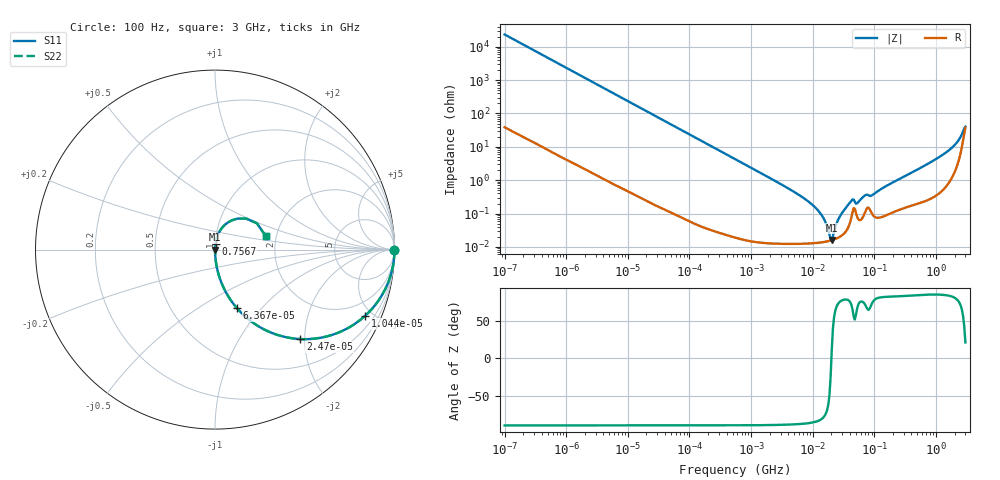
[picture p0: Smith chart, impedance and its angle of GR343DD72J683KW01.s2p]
!Murata Part Number: GR343DD72J683KW01
!These Parameters are Measured in Series Mode Connection
!Data Generated on Jan 08, 2026
!  o--ll--o
!Port1  Port2
!  o------o
!Operation Temp=25[degC], DC Bias Voltage=0[V]
!Freq. Start=100[Hz] Stop=3[GHz] 401[Steps]
# Hz S RI R 50
!Freq.(Hz) S11(Real) S11(Imag) S21(Real) S21(Imag) S12(Real) S12(Imag) S22(Real) S22(Imag)
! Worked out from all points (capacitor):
!   401 points, 100 Hz to 3 GHz, reference 50 ohm
!   read as one part in series: C = 68 nF near 109 Hz
!   lowest |Z| = 16.2 mohm at 20.36 MHz (marker M1)
!   series resonance near 20.1 MHz, so ESL is about 920 pH
!   S11 on the Smith chart (normalised r, x): 100 Hz: open; 10.44 kHz: 1.01, -4.51; 24.7 kHz: 1.00, -1.91; 63.67 kHz: 1.00, -0.74; 756.7 MHz: 1.01, +0.06; 3 GHz: 1.75, +0.29
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100  1 -0.00427  2.53e-05 0.00427  2.53e-05 0.00427  1 -0.00427
1788  0.9941 -0.0757  0.0059 0.0757  0.0059 0.0757  0.9941 -0.0757
10443  0.8349 -0.3702  0.1651 0.3702  0.1651 0.3702  0.8349 -0.3702
24699  0.4763 -0.4984  0.5237 0.4984  0.5237 0.4984  0.4763 -0.4984
31977  0.3522 -0.4766  0.6478 0.4766  0.6478 0.4766  0.3522 -0.4766
63668  0.1212 -0.3252  0.8788 0.3252  0.8788 0.3252  0.1212 -0.3252
171338  0.019 -0.1351  0.981 0.1351  0.981 0.1351  0.019 -0.1351
547723  0.00205 -0.0431  0.998 0.0431  0.998 0.0431  0.00205 -0.0431
4323298  0.00015 -0.00523  0.9998 0.00523  0.9998 0.00523  0.00015 -0.00523
9794414  0.000132 -0.00185  0.9999 0.00185  0.9999 0.00185  0.000132 -0.00185
1.442825e7  0.000139 -0.000803  0.9999 0.000803  0.9999 0.000803  0.000139 -0.000803
1.867972e7  0.000152 -0.000175  0.9998 0.000175  0.9998 0.000175  0.000152 -0.000175
2.035898e7  0.000159 3.17e-05  0.9998 -3.17e-05  0.9998 -3.17e-05  0.000159 3.17e-05
2.751729e7  0.000201 0.00079  0.9998 -0.00079  0.9998 -0.00079  0.000201 0.00079
4.231884e7  0.000761 0.00231  0.9992 -0.00231  0.9992 -0.00231  0.000761 0.00231
5.478864e7  0.00068 0.00208  0.9993 -0.00208  0.9993 -0.00208  0.00068 0.00208
7.093284e7  0.00111 0.00336  0.9989 -0.00336  0.9989 -0.00336  0.00111 0.00336
9.183415e7  0.000993 0.0034  0.999 -0.0034  0.999 -0.0034  0.000993 0.0034
1.751444e8  0.00103 0.00748  0.999 -0.00748  0.999 -0.00748  0.00103 0.00748
7.567485e8  0.00358 0.0315  0.9964 -0.0315  0.9964 -0.0315  0.00358 0.0315
2.126076e9  0.0367 0.1181  0.9633 -0.1181  0.9633 -0.1181  0.0367 0.1181
3e9  0.2818 0.0766  0.7182 -0.0766  0.7182 -0.0766  0.2818 0.0766
